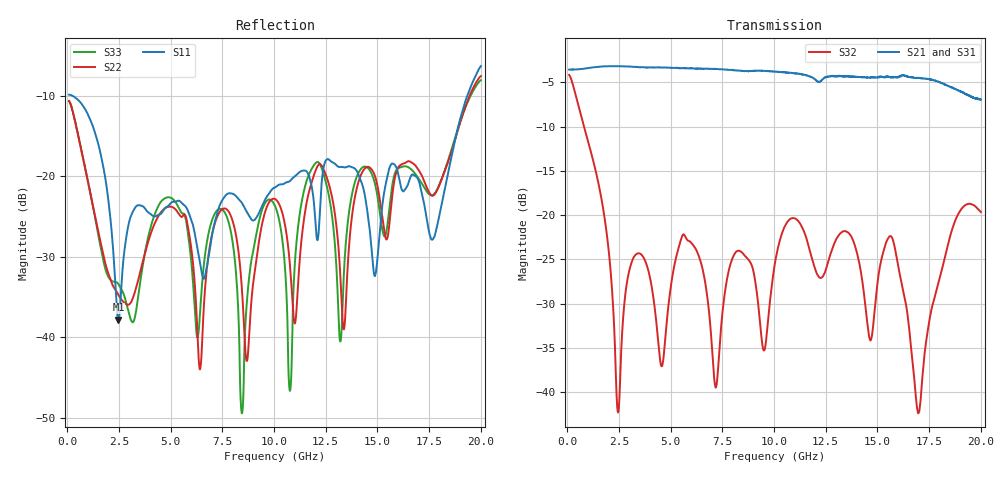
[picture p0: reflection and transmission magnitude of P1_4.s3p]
!The following data was pulled from an Agilent PNA
!This sNp file was generated from the data in the RF Test software
!NOTE:  Smoothing/Math/Corrections applied on any given trace ARE included in the data saved here
# MHz S dB R 50
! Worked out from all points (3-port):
!   6401 points, 100 MHz to 20 GHz, reference 50 ohm
!   strongest paths, dB at 100 MHz, 5.075 GHz, 10.05 GHz, 15.03 GHz, 20 GHz:
!     S21: -3.6, -3.4, -3.8, -4.4, -7.0
!     S31: -3.6, -3.4, -3.8, -4.4, -6.7
!     S32: -4.2, -27.1, -25.4, -27.3, -19.6
!   lowest |S11| = -37.8 dB at 2.482 GHz (marker M1), VSWR 1.03, Z = 49.9 + j1.28 ohm
!   |S11| at or under -10 dB: 237.3 MHz to 19.35 GHz (19.11 GHz wide, 195 % of centre)
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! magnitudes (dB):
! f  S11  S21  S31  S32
! 100 MHz  -9.9  -3.6  -3.6  -4.2
! 2.482 GHz  -37.8  -3.2  -3.2  -42.2
! 7.531 GHz  -22.8  -3.5  -3.5  -30.5
! 8.449 GHz  -23.3  -3.7  -3.8  -24.2
! 10.05 GHz  -21.4  -3.8  -3.8  -25.4
! 10.77 GHz  -20.6  -3.9  -4.0  -20.4
! 11.9 GHz  -22.6  -4.5  -4.6  -25.4
! 13.21 GHz  -18.9  -4.3  -4.3  -22.0
! 16.98 GHz  -20.4  -4.5  -4.6  -42.4
! 20 GHz  -6.4  -7.0  -6.7  -19.6
